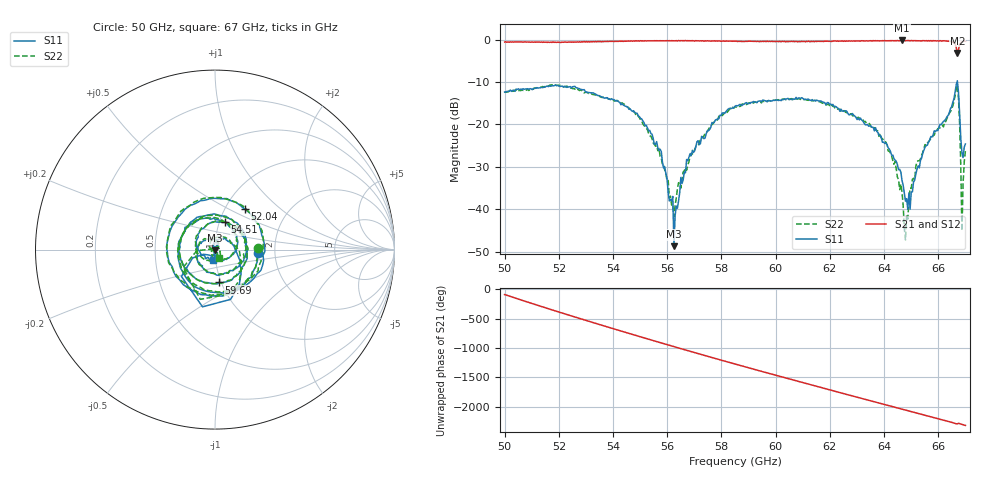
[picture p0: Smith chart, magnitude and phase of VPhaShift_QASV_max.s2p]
!Agilent Technologies,E8361A,US42410132,A.06.03.05
!Agilent E8361A: A.06.03.05
!Date: Friday, July 11, 2008 15:24:19
!Correction: S11(Full 2 Port(1,2)) S21(Full 2 Port(1,2)) S12(Full 2 Port(1,2)) S22(Full 2 Port(1,2))
!S2P File: Measurements: S11, S21, S12, S22:
# Hz S  MA  R 50
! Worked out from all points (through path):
!   401 points, 50 GHz to 67 GHz, reference 50 ohm
!   highest |S21| = -0.22 dB at 64.66 GHz (marker M1); lowest = -3.2 dB at 66.7 GHz (marker M2)
!   lowest |S11| = -48.7 dB at 56.25 GHz (marker M3), VSWR 1.01, Z = 49.8 - j0.326 ohm
!   |S11| at or under -10 dB: start of sweep to 66.69 GHz; 66.70685 GHz to end of sweep
!   |S22| runs from -47.2 to -10.7 dB; largest |S21 - S12| = 0.018
!   S11 on the Smith chart (normalised r, x): 50 GHz: 1.63, -0.06; 52.04 GHz: 1.23, +0.60; 54.51 GHz: 1.07, +0.33; 59.69 GHz: 0.98, -0.37; 67 GHz: 0.97, -0.11
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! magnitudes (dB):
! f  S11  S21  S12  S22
! 50 GHz  -12.4  -0.6  -0.5  -12.4
! 52.04 GHz  -11.1  -0.6  -0.7  -10.8
! 52.85 GHz  -11.8  -0.5  -0.5  -12.1
! 54.51 GHz  -15.8  -0.4  -0.4  -15.8
! 55.7 GHz  -26.2  -0.3  -0.3  -25.7
! 56.25 GHz  -48.7  -0.3  -0.3  -41.7
! 56.33 GHz  -39.2  -0.3  -0.3  -37.4
! 56.8 GHz  -27.7  -0.3  -0.3  -28.8
! 57.65 GHz  -19.6  -0.3  -0.4  -20.0
! 58.5 GHz  -15.7  -0.4  -0.3  -15.9
! 59.69 GHz  -14.7  -0.4  -0.5  -14.5
! 61.35 GHz  -14.2  -0.5  -0.4  -14.4
! 63.39 GHz  -20.0  -0.3  -0.3  -19.7
! 64.19 GHz  -25.8  -0.3  -0.3  -26.4
! 64.66 GHz  -33.2  -0.2  -0.3  -36.0
! 64.79 GHz  -38.1  -0.3  -0.2  -47.2
! 64.96 GHz  -40.0  -0.3  -0.3  -35.0
! 65.51 GHz  -25.4  -0.3  -0.3  -24.7
! 66.7 GHz  -9.7  -3.2  -3.2  -10.8
! 66.87 GHz  -26.7  -0.5  -0.5  -45.1
! 66.96 GHz  -25.3  -0.4  -0.4  -28.8
! 67 GHz  -24.6  -0.4  -0.5  -26.2
